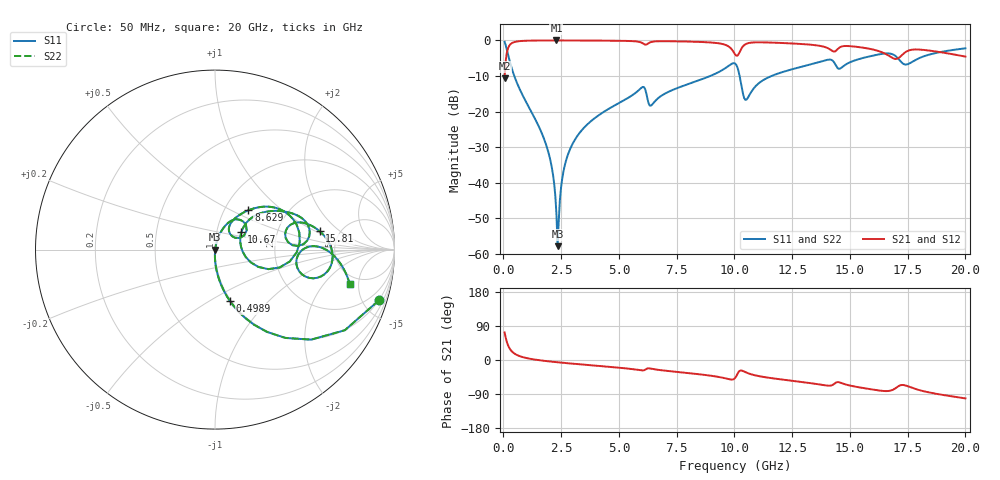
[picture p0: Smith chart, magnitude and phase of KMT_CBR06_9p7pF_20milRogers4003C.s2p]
! Data measured by Modelithics Inc. support@modelithics.com 813-866-6335
! KEMET CBR0603 9.7pF, Pad Width= 0.851mm, Pad Length= 0.64mm, Pad Gap= 0.62mm, 20mil Rogers 4003C substrate Data, January 2022
# hz S ma R 50
! 2 Port Network Data from SP1.SP block
! freq  magS11  angS11  magS21  angS21  magS12  angS12  magS22  angS22
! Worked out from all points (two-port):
!   401 points, 50 MHz to 20 GHz, reference 50 ohm
!   highest |S21| = -0.01 dB at 2.294 GHz (marker M1); lowest = -10.6 dB at 50 MHz (marker M2)
!   |S21| within 3 dB of the highest: 165 MHz to 9.94 GHz (9.775 GHz wide, 193 % of centre); 10.24 GHz to 14.25 GHz (4.008 GHz wide, 32.7 % of centre)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
!   lowest |S11| = -57.9 dB at 2.344 GHz (marker M3), VSWR 1.00, Z = 50.1 - j0.0468 ohm
!   |S11| at or under -10 dB: 469.3 MHz to 8.952 GHz (8.482 GHz wide, 180 % of centre); 10.23 GHz to 11.61 GHz (1.383 GHz wide, 12.7 % of centre)
!   |S22| runs from -57.9 to -0.4 dB; largest |S21 - S12| = 0
!   S11 on the Smith chart (normalised r, x): 50 MHz: 0.99, -6.46; 498.9 MHz: 0.99, -0.62; 8.629 GHz: 1.29, +0.62; 10.67 GHz: 1.31, +0.26; 15.81 GHz: 3.53, +1.11; 20 GHz: 4.05, -3.87
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5e7  0.9558 -17.2  0.2938 72.8  0.2938 72.8  0.9558 -17.2
2.99375e8  0.4715 -62.6  0.8812 27.4  0.8812 27.4  0.4715 -62.6
4.98875e8  0.2975 -73.8  0.954 16.0  0.954 16.0  0.2975 -73.8
1.895375e9  0.03043 -91.0  0.9983 -3.1  0.9983 -3.1  0.03043 -91.0
2.14475e9  0.01296 -89.5  0.9987 -4.8  0.9987 -4.8  0.01296 -89.5
2.294375e9  0.003596 -75.8  0.9987 -5.7  0.9987 -5.7  0.003596 -75.8
2.34425e9  0.001279 -21.4  0.9987 -6.0  0.9987 -6.0  0.001279 -21.4
2.74325e9  0.02224 78.3  0.9983 -8.3  0.9983 -8.3  0.02224 78.3
3.391625e9  0.05461 76.6  0.9969 -11.8  0.9969 -11.8  0.05461 76.6
5.985125e9  0.2174 49.4  0.9281 -27.5  0.9281 -27.5  0.2174 49.4
6.384125e9  0.1209 45.0  0.9476 -22.7  0.9476 -22.7  0.1209 45.0
6.73325e9  0.1576 58.9  0.974 -26.2  0.974 -26.2  0.1576 58.9
8.6285e9  0.2879 49.6  0.9489 -38.7  0.9489 -38.7  0.2879 49.6
9.675875e9  0.4221 32.5  0.8481 -49.3  0.8481 -49.3  0.4221 32.5
1.0025e10  0.4739 5.1  0.6388 -47.7  0.6388 -47.7  0.4739 5.1
1.0424e10  0.1539 -3.8  0.8597 -30.5  0.8597 -30.5  0.1539 -3.8
1.067338e10  0.1762 33.4  0.9258 -36.7  0.9258 -36.7  0.1762 33.4
1.336662e10  0.4664 26.1  0.8662 -61.7  0.8662 -61.7  0.4664 26.1
1.58105e10  0.5923 9.9  0.7668 -76.3  0.7668 -76.3  0.5923 9.9
1.670825e10  0.6545 -6.7  0.6026 -81.5  0.6026 -81.5  0.6545 -6.7
1.74065e10  0.4577 -8.0  0.6843 -67.2  0.6843 -67.2  0.4577 -8.0
2e10  0.7744 -14.3  0.5922 -101.3  0.5922 -101.3  0.7744 -14.3
